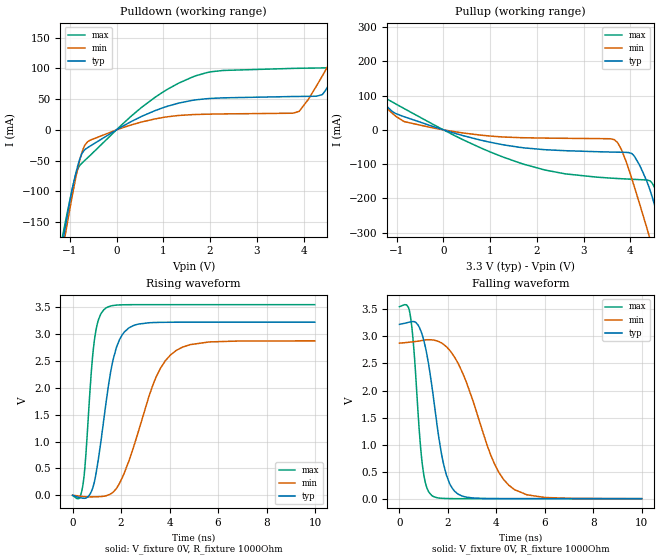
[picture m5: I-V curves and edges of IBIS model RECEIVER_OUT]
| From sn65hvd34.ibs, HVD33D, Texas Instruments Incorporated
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[Model]   RECEIVER_OUT
Model_type   Output
|Signal   R
Polarity   Non-Inverting
Enable   Active-Low
Vmeas = 1.39
Vref  = 1.65
Cref  = 15pF
| variable   typ   min   max
|   (nom PVT)   (slow PVT)   (fast PVT)
C_comp   720.5fF   606fF   852.5fF
|   typ   min   max
[Voltage Range]   3.3   3   3.6
[Temperature Range]   27   85   -40
[Pullup Reference]   3.3   3   3.6
[Pulldown Reference]   -0   -0   -0
[Power Clamp Reference]   3.3   3   3.6
[GND Clamp Reference]   -0   -0   -0
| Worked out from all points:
|   slope of the pulldown table from 0 to 0.495 V, typ, clamps not added: 24.3 ohm
|   slope of the pullup table from 0 to 0.495 V, typ, clamps not added: 25.4 ohm
|   falling waveform, V_fixture 0V, R_fixture 1000Ohm: 20-80 % time 651ps typ, 1.37ns min, 344ps max; typ from 3.22 V to 0 V
|   rising waveform, V_fixture 0V, R_fixture 1000Ohm: 20-80 % time 649ps typ, 1.29ns min, 346ps max; typ from 0 V to 3.22 V
[Pulldown]
|   Voltage   I(typ)   I(min)   I(max)
-3.3V     -1.263A    -1.197A    -1.336A
-1.171V   -193.6mA   -204.1mA   -179.8mA
-1.058V   -141.2mA   -153.8mA   -135.9mA
-844.8mV  -62.87mA   -68.11mA   -66.69mA
-617.1mV  -28.89mA   -19.25mA   -45.35mA
1.328V    43.46mA    23.39mA    75.94mA
2.036V    51.2mA     25.61mA    94.62mA
3.902V    54.34mA    29.95mA    100.2mA
4.412V    58.22mA    89.03mA    100.8mA
4.991V    148mA      167.8mA    111.4mA
5.298V    201.7mA    210.2mA    173.2mA
6.6V      433.9mA    392.3mA    469.4mA
[Pullup]
|   Voltage   I(typ)   I(min)   I(max)
-3.3V     433.9mA    350.2mA    538.7mA
-2.26V    248.1mA    205mA      299.8mA
-1.394V   97.47mA    86.65mA    111.1mA
-834.9mV  37.99mA    23.87mA    61.57mA
1.63V     -50.93mA   -22.72mA   -96.22mA
3.655V    -64.9mA    -28.57mA   -141.2mA
3.808V    -65.34mA   -57.3mA    -142.4mA
4.075V    -75.13mA   -161.7mA   -144.3mA
4.412V    -172.4mA   -313.7mA   -148.2mA
4.744V    -327.8mA   -467.9mA   -234.8mA
5.041V    -475.9mA   -606.9mA   -334.3mA
6.6V      -1.263A    -1.338A    -1.171A
[Ramp]
R_load = 1000
|   typ   min   max
dV/dt_r   1.93425/6.45713e-010   1.72556/1.2778e-009   2.13011/3.45605e-010
dV/dt_f   1.93425/6.49609e-010   1.72556/1.36431e-009   2.13011/3.42996e-010
[Falling Waveform]
V_fixture = 0V
V_fixture_min = 0V
V_fixture_max = 0V
R_fixture = 1000Ohm
C_fixture = 0F
|   Time   V(typ)   V(min)   V(max)
0s        3.224V     2.876V     3.55V
435ps     3.268V     2.895V     3.423V
600ps     3.275V     2.903V     2.737V
940ps     3.029V     2.926V     649.3mV
1.33ns    2.112V     2.937V     60.16mV
1.825ns   629.6mV    2.852V     5.078mV
2.435ns   80.74mV    2.488V     457.6uV
3.915ns   1.502mV    648.3mV    647.9nV
4.735ns   252.6uV    170.6mV    -1.234uV
9.99ns    -2.454uV   -4.286uV   -1.494uV
[Rising Waveform]
V_fixture = 0V
V_fixture_min = 0V
V_fixture_max = 0V
R_fixture = 1000Ohm
C_fixture = 0F
|   Time   V(typ)   V(min)   V(max)
0s        -2.454uV   -4.286uV   -1.494uV
415ps     -53.39mV   -22.6mV    158.2mV
890ps     230.7mV    -28.89mV   2.851V
1.07ns    690.3mV    -26.09mV   3.27V
1.34ns    1.587V     -13.3mV    3.475V
1.675ns   2.531V     59.33mV    3.535V
2.105ns   3.024V     385.5mV    3.548V
3.44ns    3.219V     2.195V     3.55V
4.28ns    3.223V     2.699V     3.55V
9.99ns    3.224V     2.876V     3.55V
